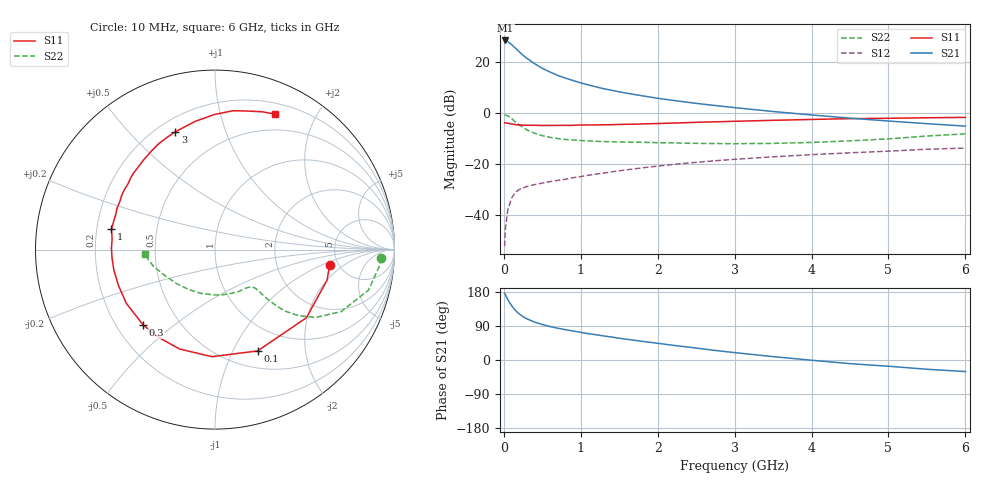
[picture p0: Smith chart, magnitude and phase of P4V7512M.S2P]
! SIEMENS Small Signal Semiconductors
! BFP182
! Si NPN RF Bipolar Junction Transistor in SOT143
! VCE = 0.75 V  IC = 12 mA
! Common Emitter S-Parameters:  March  1996
# GHz  S  MA  R  50
!  f  S11  S21  S12  S22
! GHz  MAG  ANG  MAG  ANG  MAG  ANG  MAG  ANG
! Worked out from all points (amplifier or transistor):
!   36 points, 10 MHz to 6 GHz, reference 50 ohm
!   highest |S21| = 28.4 dB at 20 MHz (marker M1)
!   |S21| within 3 dB of that: start of sweep to 150 MHz
!   unconditionally stable (mu >= 1): 617.7 MHz to end of sweep
!   at 250 MHz: K = 0.51, MSG = 25.9 dB, |S12| = -29.3 dB
!   at 1.4 GHz: K = 1.44, MAG = 12.0 dB, |S12| = -23.0 dB
!   at 6 GHz: K = 1.22, MAG = 1.5 dB, |S12| = -13.7 dB
!   S11 on the Smith chart (normalised r, x): 10 MHz: 4.26, -1.23; 100 MHz: 0.69, -1.25; 300 MHz: 0.31, -0.39; 1 GHz: 0.26, +0.09; 3 GHz: 0.27, +0.68; 6 GHz: 0.32, +1.49
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0.01  0.6446 -7.5  26.38 176.1  0.0025 83.0  0.928 -2.9
0.02  0.6472 -15.2  26.39 172.2  0.0054 80.2  0.9191 -6.0
0.05  0.6353 -36.7  25.3 160.1  0.0125 75.1  0.8844 -14.8
0.1  0.6124 -67.2  22 143.6  0.0217 60.5  0.7828 -26.2
0.15  0.5968 -91.6  18.69 130.9  0.0281 51.7  0.6763 -34.0
0.2  0.588 -109.6  15.88 121.5  0.0321 46.8  0.592 -38.4
0.25  0.5812 -122.9  13.53 114.1  0.0344 43.2  0.5235 -41.1
0.3  0.5801 -133.6  11.78 108.6  0.0368 40.7  0.4705 -42.4
0.4  0.5777 -148.7  9.27 100.0  0.04 39.6  0.4033 -43.3
0.5  0.5739 -159.8  7.534 93.7  0.0428 39.3  0.3626 -43.5
0.6  0.5749 -168.6  6.377 88.3  0.0458 39.8  0.3364 -43.5
0.7  0.5755 -175.0  5.469 83.9  0.0484 40.7  0.3183 -43.7
0.8  0.5772 179.2  4.845 79.9  0.0509 41.5  0.3054 -44.1
1  0.5877 168.9  3.906 72.9  0.0574 42.9  0.2913 -45.7
1.1  0.586 164.7  3.565 69.5  0.0611 43.7  0.2863 -47.0
1.5  0.6014 149.9  2.612 57.4  0.0744 44.0  0.2732 -53.0
2.2  0.6385 128.6  1.776 38.8  0.0991 41.6  0.2618 -68.3
3  0.6927 108.6  1.282 19.5  0.1251 35.7  0.2525 -91.2
3.5  0.7233 98.7  1.076 8.9  0.1399 31.7  0.2562 -107.7
4.5  0.7802 82.6  0.798 -9.6  0.1676 23.1  0.2873 -139.4
5.5  0.8117 71.1  0.622 -24.4  0.1967 14.9  0.3566 -165.1
6  0.8256 66.0  0.557 -30.5  0.2076 9.7  0.3929 -176.2
